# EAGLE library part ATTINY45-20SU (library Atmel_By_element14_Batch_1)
8-bit Microcontroller with 4 Bytes In-System Programmable Flash
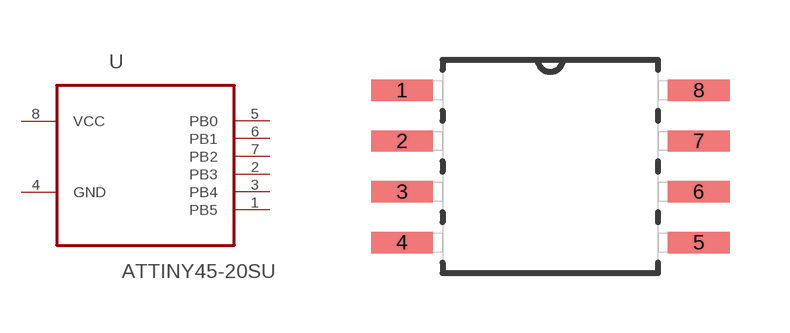
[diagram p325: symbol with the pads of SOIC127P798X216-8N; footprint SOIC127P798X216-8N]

Designator prefix U

## ATTINY45-20SU (MPN: ATTINY45-20SU; OC_FARNELL: 1288353; OC_NEWARK: 23M5073; PACKAGE: SOIC-8; SUPPLIER: Atmel)  [SOIC127P798X216-8N]
1  PB5
2  PB3
3  PB4
4  GND  pas
5  PB0
6  PB1
7  PB2
8  VCC  pwr

## Footprint SOIC127P798X216-8N (pad centres in mm)
smd 1.549 x 0.533: 1 -3.708,1.905; 2 -3.708,0.635; 3 -3.708,-0.635; 4 -3.708,-1.905; 5 3.708,-1.905; 6 3.708,-0.635; 7 3.708,0.635; 8 3.708,1.905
